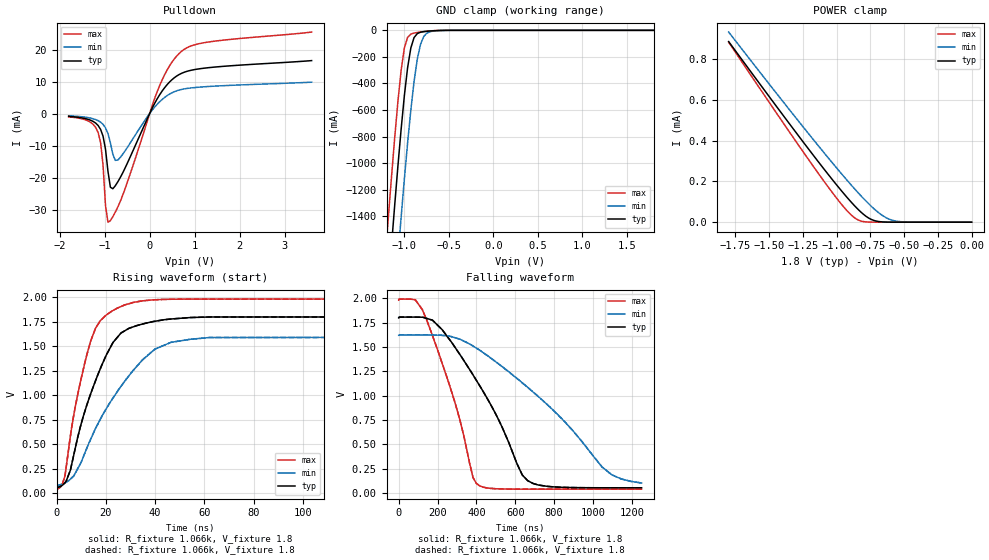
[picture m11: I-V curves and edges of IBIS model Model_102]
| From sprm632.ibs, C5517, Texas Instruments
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| Model based on original model for BI2C33T
|   Sub model BI2C33T_IND_1P8
[model]   Model_102
|[Description]  [1.8V-I/O_OPEN_DRAIN-X-X]
|   , ,
|[Input Load]
|[Output Drive]
|Voltage   1.8V
|Mode   I/O_OPEN_DRAIN
Model_type   I/O_open_drain
Polarity   Non-Inverting
Enable   Active-Low
Vinl =  0.54
Vinh =  1.26
Cref =  400pF
Rref =  528
Vref =  1.8V
Vmeas =  0.9
C_comp   2.7761451p   2.343455p   3.4415601p
[Model Spec]
Vinl   0.54   0.486   0.594
Vinh   1.26   1.134   1.386
[Temperature Range]   25   105   -40
[Voltage Range]   1.8   1.62   1.98
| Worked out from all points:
|   slope of the pulldown table from 0 to 0.27 V, typ, clamps not added: 39.3 ohm
|   GND clamp passes 1 mA (typ) near -0.59 V on its own axis
|   rising waveform, R_fixture 1.066k, V_fixture 1.8: 20-80 % time 14ns typ, 22.1ns min, 9.66ns max; typ from 0.055 V to 1.8 V
|   rising waveform, R_fixture 1.066k, V_fixture 1.8: 20-80 % time 14ns typ, 22.1ns min, 9.66ns max; typ from 0.055 V to 1.8 V
|   falling waveform, R_fixture 1.066k, V_fixture 1.8: 20-80 % time 283ns typ, 470ns min, 174ns max; typ from 1.8 V to 0.055 V
|   falling waveform, R_fixture 1.066k, V_fixture 1.8: 20-80 % time 283ns typ, 470ns min, 174ns max; typ from 1.8 V to 0.055 V
[POWER_clamp]
-1.8V     886.4uA    933.1uA    883.3uA
-1.4V     527.6uA    594.1uA    491.3uA
-1.127V   289.4uA    368.3uA    231.7uA
-963.6mV  153.6uA    237.5uA    87.55uA
-872.7mV  84.52uA    168.1uA    24.38uA
-818.2mV  48.44uA    128.4uA    5.356uA
-745.5mV  14.21uA    79.37uA    311.3nA
-709.1mV  5.812uA    57.5uA     56.41nA
-654.5mV  1.198uA    30.21uA    4.358nA
-581.8mV  94.65nA    8.572uA    266.5pA
-472.7mV  1.812nA    662.5nA    129.2pA
0V        140.3pA    2.174nA    89.79pA
[Pulldown]
-1.8V     -888.4uA   -690.4uA   -1.029mA
-1.145V   -3.74mA    -2.222mA   -5.934mA
-1.091V   -4.938mA   -2.689mA   -9.018mA
-1.036V   -7.046mA   -3.375mA   -16.04mA
-981.8mV  -11.08mA   -4.445mA   -28.66mA
-927.3mV  -17.97mA   -6.221mA   -33.93mA
-872.7mV  -23.02mA   -9.142mA   -33.44mA
-709.1mV  -21.36mA   -14.53mA   -29.23mA
163.6mV   4.505mA    2.839mA    6.699mA
654.5mV   12.17mA    7.339mA    18.75mA
1.255V    14.24mA    8.398mA    22.22mA
3.6V      16.53mA    9.79mA     25.44mA
[GND_clamp]
-1.8V     -7.773A    -8.459A    -7.277A
-1.218V   -2.273A    -2.982A    -1.749A
-1.182V   -1.949A    -2.656A    -1.427A
-1.145V   -1.632A    -2.335A    -1.114A
-1.109V   -1.323A    -2.019A    -815.7mA
-1.036V   -746.7mA   -1.409A    -303mA
-1V       -493.2mA   -1.121A    -133.4mA
-927.3mV  -133.1mA   -600.8mA   -28.5mA
-854.5mV  -24.65mA   -217mA     -16.09mA
-818.2mV  -14.19mA   -105.1mA   -12.49mA
-709.1mV  -4.932mA   -9.826mA   -4.338mA
1.8V      140.3pA    2.551nA    74.6pA
[Ramp]
dV/dt_f 0.41925174/0.4235738u 0.25012434/0.64769712u 0.63452282/0.26961151u
dV/dt_r 3.8786023m/4.7653768n 2.4355876m/4.9752319n 5.8608085m/3.9341721n
R_load = 50
[Rising Waveform]
R_fixture = 1.066k
V_fixture = 1.8
V_fixture_min = 1.62
V_fixture_max = 1.98
0s        55.3mV     78.77mV    41.55mV
3.436ns   108.2mV    106mV      178.6mV
5.628ns   235.5mV    144.4mV    582.9mV
8.892ns   599.9mV    264.4mV    1.042V
15.84ns   1.149V     661.9mV    1.684V
22.89ns   1.537V     970.9mV    1.864V
26.15ns   1.634V     1.09V      1.905V
39.19ns   1.751V     1.454V     1.972V
61.98ns   1.798V     1.588V     1.981V
1.25us    1.8V       1.62V      1.98V
[Rising Waveform]
R_fixture = 1.066k
V_fixture = 1.8
V_fixture_min = 1.62
V_fixture_max = 1.98
0s        55.3mV     78.77mV    41.55mV
3.436ns   108.2mV    106mV      178.6mV
5.628ns   235.5mV    144.4mV    582.9mV
8.892ns   599.9mV    264.4mV    1.042V
15.84ns   1.149V     661.9mV    1.684V
22.89ns   1.537V     970.9mV    1.864V
26.15ns   1.634V     1.09V      1.905V
39.19ns   1.751V     1.454V     1.972V
61.98ns   1.798V     1.588V     1.981V
1.25us    1.8V       1.62V      1.98V
[Falling Waveform]
R_fixture = 1.066k
V_fixture = 1.8
V_fixture_min = 1.62
V_fixture_max = 1.98
0s        1.8V       1.621V     1.981V
85.48ns   1.808V     1.625V     1.986V
121.8ns   1.806V     1.625V     1.885V
173.7ns   1.776V     1.624V     1.619V
287.1ns   1.506V     1.598V     947mV
382.6ns   1.214V     1.51V      160.2mV
399.8ns   1.158V     1.489V     99.74mV
664.2ns   127.4mV    1.086V     40.75mV
1.046us   55.06mV    269.5mV    40.78mV
1.25us    54.89mV    104.6mV    40.78mV
[Falling Waveform]
R_fixture = 1.066k
V_fixture = 1.8
V_fixture_min = 1.62
V_fixture_max = 1.98
0s        1.8V       1.621V     1.981V
85.48ns   1.808V     1.625V     1.986V
121.8ns   1.806V     1.625V     1.885V
173.7ns   1.776V     1.624V     1.619V
287.1ns   1.506V     1.598V     947mV
382.6ns   1.214V     1.51V      160.2mV
399.8ns   1.158V     1.489V     99.74mV
664.2ns   127.4mV    1.086V     40.75mV
1.046us   55.06mV    269.5mV    40.78mV
1.25us    54.89mV    104.6mV    40.78mV
